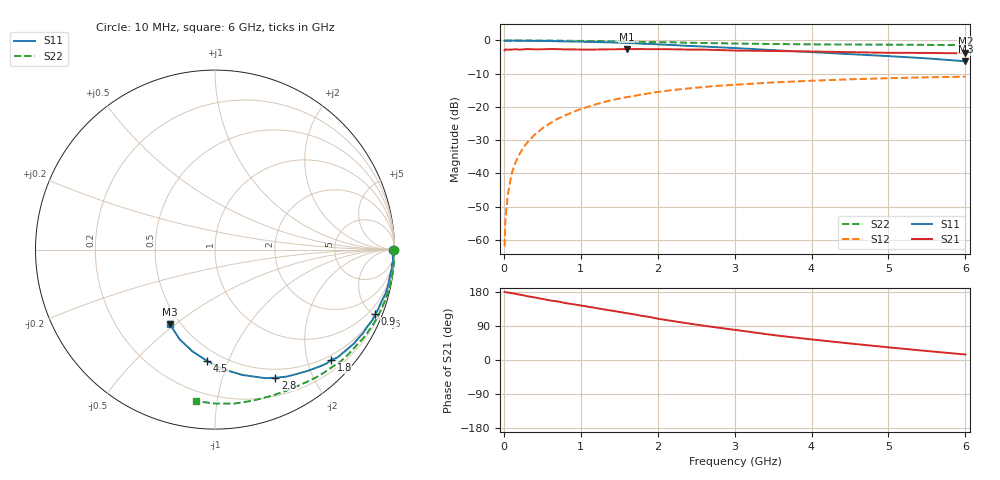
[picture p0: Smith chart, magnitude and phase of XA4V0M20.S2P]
! SIEMENS Discrete & RF Semiconductors
! BFY180
! Si NPN RF Bipolar Junction Transistor in MICRO-X
! VCE = 4 V  IC = 0.2 mA
! Common Emitter S-Parameters:  May  1997
# GHz  S  MA  R  50
!  f  S11  S21  S12  S22
! GHz  MAG  ANG  MAG  ANG  MAG  ANG  MAG  ANG
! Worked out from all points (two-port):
!   36 points, 10 MHz to 6 GHz, reference 50 ohm
!   highest |S21| = -2.57 dB at 1.6 GHz (marker M1); lowest = -3.9 dB at 6 GHz (marker M2)
!   |S21| within 3 dB of the highest: start of sweep to end of sweep
!   lowest |S11| = -6.3 dB at 6 GHz (marker M3), VSWR 2.89, Z = 22 - j23.9 ohm
!   |S11| at or under -10 dB: nowhere
!   |S22| runs from -1.4 to 0.0 dB; largest |S21 - S12| = 0.74
!   S11 on the Smith chart (normalised r, x): 10 MHz: open; 900 MHz: 0.52, -5.09; 1.8 GHz: 0.40, -2.44; 2.8 GHz: 0.40, -1.50; 4.5 GHz: 0.42, -0.84; 6 GHz: 0.44, -0.48
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0.01  0.9935 -0.2  0.709 179.9  0.0008 81.4  0.9991 -0.2
0.02  0.9938 -0.4  0.734 178.9  0.002 97.7  0.9999 -0.4
0.05  0.9911 -1.1  0.726 178.3  0.0046 86.2  0.9981 -1.0
0.1  0.9917 -2.5  0.729 176.4  0.0098 89.6  0.9961 -2.0
0.15  0.9954 -3.9  0.737 174.6  0.0144 86.9  0.9999 -3.0
0.2  0.989 -4.8  0.729 172.6  0.0191 85.7  0.9993 -4.0
0.25  0.9912 -6.2  0.732 171.1  0.0241 85.0  0.9994 -5.0
0.3  0.9877 -7.3  0.743 168.5  0.0287 83.6  0.9974 -5.9
0.4  0.9852 -9.6  0.735 165.1  0.0381 82.1  0.9979 -7.9
0.5  0.9847 -12.2  0.736 161.3  0.0474 79.6  0.9962 -9.9
0.7  0.972 -17.0  0.741 154.6  0.0662 74.8  0.9924 -13.8
0.9  0.9628 -22.0  0.733 147.2  0.0838 70.6  0.987 -17.8
1.1  0.9514 -26.7  0.727 140.5  0.1008 66.6  0.9803 -21.7
1.6  0.9161 -38.9  0.744 123.5  0.1402 56.3  0.9609 -31.3
1.8  0.8922 -43.6  0.741 116.3  0.1543 52.5  0.9508 -34.8
2.2  0.852 -52.3  0.736 102.7  0.1794 44.7  0.9361 -42.0
2.8  0.7886 -64.8  0.717 84.9  0.2083 34.7  0.908 -51.5
3.5  0.7149 -77.7  0.694 65.8  0.2334 24.5  0.8843 -61.7
4  0.6679 -86.2  0.682 54.3  0.2477 17.9  0.8737 -68.8
4.5  0.6221 -94.0  0.666 43.6  0.26 11.8  0.8678 -75.8
5.5  0.5371 -111.6  0.649 23.7  0.2785 0.1  0.8576 -90.2
6  0.4858 -121.1  0.639 14.5  0.2851 -5.9  0.8502 -97.3
